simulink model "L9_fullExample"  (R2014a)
settings: Solver=ode45  StartTime=0.0  StopTime=tend  RelTol=1e-3
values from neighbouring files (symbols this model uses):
  A = [0 1; 0 0]    [L9.m]    (also in L9_LandObs_script.m; L9_fullExample_script.m; L9_onlyL_script.m)
  Aob = Phi-Gamma*L-K*C    [L9_LandObs_script.m]    (also in L9_fullExample_script.m = [ Phi-Gamma*L-K*C, zeros(size(A,1),1))
  B = [0; 1]    [L9.m]    (also in L9_LandObs_script.m; L9_fullExample_script.m; L9_onlyL_script.m)
  Bob = K    [L9_LandObs_script.m]    (also in L9_fullExample_script.m = Ke)
  C = [1, 0]    [L9.m]    (also in L9_LandObs_script.m; L9_fullExample_script.m; L9_onlyL_script.m)
  Cob = eye(size(Aob))    [L9_LandObs_script.m]    (also in L9_fullExample_script.m)
  Cobw = Cob(size(Phi,1)+1:end,:)    [L9_fullExample_script.m]
  Cobx = Cob(1:size(Phi,1),:)    [L9_fullExample_script.m]
  Cx = eye(size(A))    [L9.m]    (also in L9_LandObs_script.m; L9_fullExample_script.m; L9_onlyL_script.m)
  Dob = zeros(size(Cob,1),size(Bob,2))    [L9_LandObs_script.m]    (also in L9_fullExample_script.m)
  Dx = zeros(size(Cx,1),size(B,2))    [L9.m]    (also in L9_LandObs_script.m; L9_fullExample_script.m; L9_onlyL_script.m)
  h = h3    (= 0.5)    [L9.m]    (also in L9_LandObs_script.m = 0.44; L9_fullExample_script.m = 0.44; L9_onlyL_script.m = 0.44)
  Lob = [ L, 1]    [L9_fullExample_script.m]
  x0 = [1;1]    [L9.m]    (also in L9_LandObs_script.m; L9_fullExample_script.m; L9_onlyL_script.m)
libraries: simulink x1

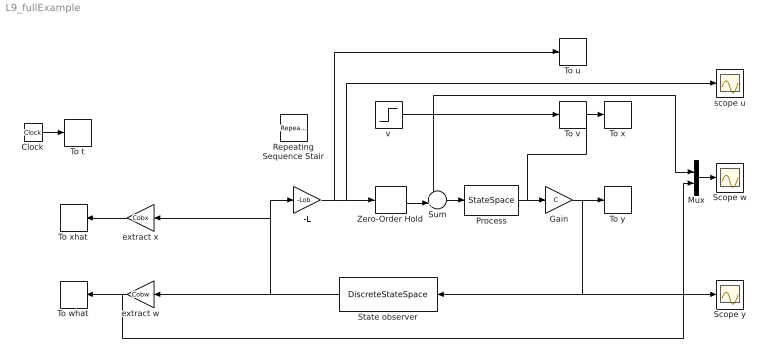
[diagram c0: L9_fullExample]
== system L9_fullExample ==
  -L : Gain  Gain=-Lob  Multiplication=Matrix(K*u)  SampleTime=h
  Clock : Clock
  Gain : Gain  Gain=C  Multiplication=Matrix(K*u)
  Mux : Mux  Inputs=2
  Process : StateSpace  A=A  B=B  C=Cx  D=Dx  X0=x0
  Repeating Sequence Stair : simulink/Sources/Repeating Sequence Stair  OutValues=[0 0 0 0 0 0 0 0 0 0 0 0 0 0 -0.5 ].'  tsamp=1  OutMin=[]  OutMax=[]  OutDataTypeStr=double  OutputDataTypeScalingMode=double  OutDataType=fixdt(0,8)  ConRadixGroup=Best Precision: Vector-wise  OutScaling=2^-12
  Scope w : Scope
  Scope y : Scope
  State observer : DiscreteStateSpace  A=Aob  B=Bob  C=Cob  D=Dob  SampleTime=h
  Sum : Sum  Inputs=++|
  To t : ToWorkspace  VariableName=t  SampleTime=h
  To u : ToWorkspace  VariableName=u  SampleTime=h
  To v : ToWorkspace  VariableName=v  SaveFormat=Structure With Time  SampleTime=-1
  To what : ToWorkspace  VariableName=what  SampleTime=h
  To x : ToWorkspace  VariableName=x  SaveFormat=Structure With Time  SampleTime=-1
  To xhat : ToWorkspace  VariableName=xhat  SampleTime=h
  To y : ToWorkspace  VariableName=y  SaveFormat=Structure With Time  SampleTime=-1
  Zero-Order Hold : ZeroOrderHold  SampleTime=h
  extract w : Gain  Gain=Cobw  Multiplication=Matrix(K*u)  SampleTime=h
  extract x : Gain  Gain=Cobx  Multiplication=Matrix(K*u)  SampleTime=h
  scope u : Scope
  v : Step  Time=25  After=-0.5  SampleTime=0
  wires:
  -L/1 -> To u/1, scope u/1, Zero-Order Hold/1
  Clock/1 -> To t/1
  Process/1 -> To x/1, Gain/1
  State observer/1 -> extract w/1, extract x/1, -L/1
  Sum/1 -> Process/1
  Zero-Order Hold/1 -> Sum/2
  extract x/1 -> To xhat/1
  extract w/1 -> Mux/2, To what/1
  Mux/1 -> Scope w/1
  v/1 -> Sum/1, Mux/1, To v/1
  Gain/1 -> Scope y/1, State observer/1, To y/1
